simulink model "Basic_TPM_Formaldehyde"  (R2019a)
settings: Solver=ode15s  StartTime=0.0  StopTime=tend  RelTol=1e-3
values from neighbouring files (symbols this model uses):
  c_MeOH_0 = m_MeOH_sp_0/(m_MeOH_sp_0+m_air_sp_0)    [Mixer_script.m]
  comp_actuator_0 = [z0actuator,comp_w0]    [Compressor_script.m]
  comp_actuator_par = [comp_act_Ga;comp_act_tau;comp_act_zeta]    [Compressor_script.m]
  comp_deltaP = 2.1    [Compressor_script.m]
  comp_p1 = [a0,a1,a2,a3,b0,b1,b2,c0,c1,c2]    [Compressor_script.m]
  comp_p2 = [rho_a, kappa_a, cp_a, R_a, T_amb, d_c]    [Compressor_script.m]
  I_0_compressor = 0.39275    [Compressor_script.m]
  I_0_valve = valve_z0/valve_act_Ga    (= 0.7)    [Valve_script.m]
  Kc_comp = tau_compfotd/(K_compfotd*(tauc_comp+theta_compfotd))    [Compressor_script.m]
  Kc_mtot_air = tau_mtot_air/(K_mtot_air*(tauc_mtot_air+theta_mtot_air))    (= 0.512420362808)    [Basic_outer_PID_script.m]
  Kc_valve = tau_valvefotd/(K_valvefotd*(tauc_valve+theta_valvefotd))    [Valve_script.m]
  Kc_x_MeOH = tau_x_MeOH/(K_x_MeOH*(tauc_x_MeOH+theta_x_MeOH))    (= 21795.1661228)    [Basic_outer_PID_script.m]
  KI_comp = Kc_comp/tauI_comp    [Compressor_script.m]
  KI_mtot_air = Kc_mtot_air/tauI_mtot_air    [Basic_outer_PID_script.m]
  KI_valve = Kc_valve/tauI_valve    [Valve_script.m]
  KI_x_MeOH = Kc_x_MeOH/tauI_x_MeOH    [Basic_outer_PID_script.m]
  m_air_sp_0 = 23920    [Compressor_script.m]
  m_air_sp_step = m_air_sp_0*0*0.05    [main_basicTPM_formaldehyde.m]    (also in main_VPC_formaldehyde.m = m_air_sp_0*0; main_basic_formaldehyde.m = m_air_sp_0*0; main_SRC_formaldehyde.m = m_air_sp_0*0)
  m_air_sp_step_time = 20    [main_basicTPM_formaldehyde.m]    (also in main_VPC_formaldehyde.m; main_basic_formaldehyde.m; main_SRC_formaldehyde.m)
  m_MeOH_sp_0 = 2940    [Valve_script.m]
  m_MeOH_sp_step = -m_MeOH_sp_0*0.1    [main_basicTPM_formaldehyde.m]    (also in main_VPC_formaldehyde.m; main_basic_formaldehyde.m; main_SRC_formaldehyde.m)
  m_MeOH_sp_step_time = 20    [main_basicTPM_formaldehyde.m]    (also in main_VPC_formaldehyde.m; main_basic_formaldehyde.m; main_SRC_formaldehyde.m)
  m_tot_sp_0 = m_air_sp_0+m_MeOH_sp_0    [main_basicTPM_formaldehyde.m]    (also in main_VPC_formaldehyde.m; main_basic_formaldehyde.m; main_SRC_formaldehyde.m)
  m_tot_sp_step1 = 0*m_tot_sp_0*0.15    [main_basicTPM_formaldehyde.m]    (also in main_VPC_formaldehyde.m; main_basic_formaldehyde.m; main_SRC_formaldehyde.m)
  m_tot_sp_step2 = 1*m_tot_sp_0*0.10    [main_basicTPM_formaldehyde.m]    (also in main_VPC_formaldehyde.m; main_basic_formaldehyde.m; main_SRC_formaldehyde.m)
  m_tot_sp_step3 = -1*(m_tot_sp_step2+m_tot_sp_step1)    [main_basicTPM_formaldehyde.m]    (also in main_VPC_formaldehyde.m = 0*(m_tot_sp_step2+m_tot_sp_step1); main_basic_formaldehyde.m; main_SRC_formaldehyde.m)
  m_tot_sp_step_t1 = 20    [main_basicTPM_formaldehyde.m]    (also in main_VPC_formaldehyde.m; main_basic_formaldehyde.m; main_SRC_formaldehyde.m)
  m_tot_sp_step_t2 = 30    [main_basicTPM_formaldehyde.m]    (also in main_VPC_formaldehyde.m; main_basic_formaldehyde.m; main_SRC_formaldehyde.m)
  m_tot_sp_step_t3 = 70    [main_basicTPM_formaldehyde.m]    (also in main_VPC_formaldehyde.m = 60; main_basic_formaldehyde.m; main_SRC_formaldehyde.m)
  max_air_PI = mair_max-m_air_sp_0    [Basic_outer_PID_script.m]
  max_MeOH_PI = m_MeOH_max-m_MeOH_sp_0    [Basic_outer_PID_script.m]
  min_air_PI = mair_min-m_air_sp_0    [Basic_outer_PID_script.m]
  min_MeOH_PI = m_MeOH_min-m_MeOH_sp_0    [Basic_outer_PID_script.m]
  N_cmax = 10048    [Compressor_script.m]
  N_cmin = 7500    [Compressor_script.m]
  p_mix = [MW_MeOH;MW_air;rho_MeOH;rho_a;V_mixer]    [Mixer_script.m]
  PI_comp_max = 0.2    [Compressor_script.m]
  PI_comp_min = -I_0_compressor    (= -0.39275)    [Compressor_script.m]
  valve_actuator_0 = [valve_z0 valve_w0]    [Valve_script.m]
  valve_actuator_par = [valve_act_Ga;valve_act_tau;valve_act_zeta]    [Valve_script.m]
  valve_Cv = m_MeOH_max/sqrt(valve_delta_p)    [Valve_script.m]
  valve_delta_p = 0.5    [Valve_script.m]
  valve_type = 3    [Valve_script.m]
  x_MeOH_sp_step1 = 1*-0.005    (= -0.005)    [main_basicTPM_formaldehyde.m]    (also in main_VPC_formaldehyde.m; main_basic_formaldehyde.m; main_SRC_formaldehyde.m)
  x_MeOH_sp_step2 = 0*-0.005    (= 0)    [main_basicTPM_formaldehyde.m]    (also in main_VPC_formaldehyde.m; main_basic_formaldehyde.m; main_SRC_formaldehyde.m)
  x_MeOH_sp_step3 = 0*+0.01    (= 0)    [main_basicTPM_formaldehyde.m]    (also in main_VPC_formaldehyde.m; main_basic_formaldehyde.m; main_SRC_formaldehyde.m)
  x_MeOH_sp_step_t1 = 10    [main_basicTPM_formaldehyde.m]    (also in main_VPC_formaldehyde.m; main_basic_formaldehyde.m; main_SRC_formaldehyde.m)
  x_MeOH_sp_step_t2 = 40    [main_basicTPM_formaldehyde.m]    (also in main_VPC_formaldehyde.m; main_basic_formaldehyde.m; main_SRC_formaldehyde.m)
  x_MeOH_sp_step_t3 = 70    [main_basicTPM_formaldehyde.m]    (also in main_VPC_formaldehyde.m = 60; main_basic_formaldehyde.m; main_SRC_formaldehyde.m)
  x_MeOHsp_0 = 0.1    [main_basicTPM_formaldehyde.m]    (also in main_VPC_formaldehyde.m; main_basic_formaldehyde.m; main_SRC_formaldehyde.m)
undefined symbols (not defined in the file or in its folder): actuator, compressor, mixerMeOH_O2_dynamic, mixerMeOH_O2_ss, valve
libraries: simulink x4

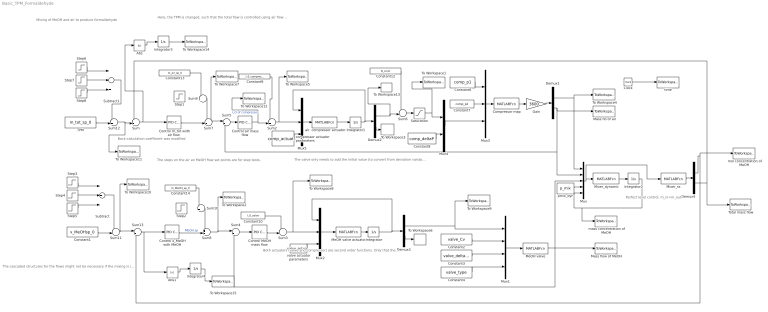
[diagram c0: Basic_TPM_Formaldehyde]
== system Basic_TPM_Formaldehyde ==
  note: Mixing of MeOH and air to produce formaldehyde
  note: The cascaded structures for the flows might not be necessary if the mixing is instantaneous. I just added them to have a general structure. I also added a small residence time in the tank.
  note: Both actuators (valve and compressor) are second order functions. Only that the time constants and the damping factors are different.
  note: The valve only needs to add the initial value (to convert from deviation variables to actual variables "once" before the actuator. The compressor also needs it before the actuator because the range does not start in 0. (Maybe there is a better way to do this).
  note: Perfect level control. m_in=m_out
  note: The steps on the air an MeOH flow set points are for step tests.
  note: Here, the TPM is changed, such that the total flow is controlled using air flow and the concentration is set by the flow of MeOH
  note: Back-calculation coefficient was modified
  Abs : Abs
  Abs1 : Abs
  Clock : Clock
  Compressor map : MATLABFcn  MATLABFcn=compressor(u(1:10),u(11:16),u(17:18))  OutputDimensions=2
  Constant1 : Constant  Value=x_MeOHsp_0
  Constant10 : Constant  Value=I_0_valve
  Constant12 : Constant  Value=N_cmin
  Constant13 : Constant  Value=m_air_sp_0
  Constant14 : Constant  Value=m_MeOH_sp_0
  Constant2 : Constant  Value=valve_Cv
  Constant3 : Constant  Value=valve_delta_p
  Constant4 : Constant  Value=valve_type
  Constant6 : Constant  Value=comp_p1
  Constant7 : Constant  Value=comp_p2
  Constant8 : Constant  Value=comp_deltaP
  Constant9 : Constant  Value=I_0_compressor
  Control MeOH mass flow : simulink/Continuous/PID Controller  Controller=PI  Form=Parallel  TimeDomain=Continuous-time  SampleTime=-1  IntegratorMethod=Forward Euler  FilterMethod=Forward Euler  ControllerParametersSource=internal  P=Kc_valve  I=KI_valve  D=0  UseFilter=on  N=100  TunerSelectOption=Transfer Function Based (PID Tuner App)  InitialConditionSource=internal  InitialConditionForIntegrator=0  InitialConditionForFilter=0  DifferentiatorICPrevScaledInput=0  ExternalReset=none  TrackingMode=off  Kt=1  LimitOutput=on  UpperSaturationLimit=1-I_0_valve  LowerSaturationLimit=-I_0_valve  LinearizeAsGain=on  AntiWindupMode=back-calculation  Kb=1  POutMin=[]  POutMax=[]  IOutMin=[]  IOutMax=[]  DOutMin=[]  DOutMax=[]  NOutMin=[]  NOutMax=[]  SumOutMin=[]  SumOutMax=[]  SaturationOutMin=[]  SaturationOutMax=[]  PParamMin=[]  PParamMax=[]  IParamMin=[]  IParamMax=[]  DParamMin=[]  DParamMax=[]  NParamMin=[]  NParamMax=[]  KbParamMin=[]  KbParamMax=[]  KtParamMin=[]  KtParamMax=[]  KbOutMin=[]  KbOutMax=[]  KtOutMin=[]  KtOutMax=[]  IntegratorOutMin=[]  IntegratorOutMax=[]  FilterOutMin=[]  FilterOutMax=[]  SumI1OutMin=[]  SumI1OutMax=[]  SumI2OutMin=[]  SumI2OutMax=[]  SumI3OutMin=[]  SumI3OutMax=[]  SumI4OutMin=[]  SumI4OutMax=[]  SumDOutMin=[]  SumDOutMax=[]  DifferentiatorOutMin=[]  DifferentiatorOutMax=[]  FilterDiffOutCoefMin=[]  FilterDiffOutCoefMax=[]  ReciprocalOutMin=[]  ReciprocalOutMax=[]  SumDenOutMin=[]  SumDenOutMax=[]  SumNumOutMin=[]  SumNumOutMax=[]  DivideOutMin=[]  DivideOutMax=[]  IntegratorContinuousStateAttributes=''  IntegratorStateMustResolveToSignalObject=off  IntegratorRTWStateStorageClass=Auto  FilterContinuousStateAttributes=''  FilterStateMustResolveToSignalObject=off  FilterRTWStateStorageClass=Auto  ParallelPVariant=InternalParameters  IdealPVariant=Disabled  IVariant=InternalParameters  DVariant=Disabled  IntegratorVariant=Continuous  SatVariant=Enabled  AWVariant=BackCalculation  PCopyVariant=Disabled  TRVariant=Disabled  FdbkBlocksVariant=Forward  IdealPFdbkVariant=Disabled  SatFdbkVariant=Disabled  DerivativeFilterVariant=Disabled  NVariant=Disabled  NCopyVariant=Disabled_SignalSpec  FilterICVariant=Disabled  IntegratorICVariant=InternalICs  ExternalResetVariant=Disabled  TRSumVariant=Passthrough  SumFdbkVariant=Disabled  SumVariant=Sum_PI
  Control air mass flow : simulink/Continuous/PID Controller  Controller=PI  Form=Parallel  TimeDomain=Continuous-time  SampleTime=-1  IntegratorMethod=Forward Euler  FilterMethod=Forward Euler  ControllerParametersSource=internal  P=Kc_comp  I=KI_comp  D=0  UseFilter=on  N=100  TunerSelectOption=Transfer Function Based (PID Tuner App)  InitialConditionSource=internal  InitialConditionForIntegrator=0  InitialConditionForFilter=0  DifferentiatorICPrevScaledInput=0  ExternalReset=none  TrackingMode=off  Kt=1  LimitOutput=on  UpperSaturationLimit=PI_comp_max  LowerSaturationLimit=PI_comp_min  LinearizeAsGain=on  AntiWindupMode=back-calculation  Kb=1  POutMin=[]  POutMax=[]  IOutMin=[]  IOutMax=[]  DOutMin=[]  DOutMax=[]  NOutMin=[]  NOutMax=[]  SumOutMin=[]  SumOutMax=[]  SaturationOutMin=[]  SaturationOutMax=[]  PParamMin=[]  PParamMax=[]  IParamMin=[]  IParamMax=[]  DParamMin=[]  DParamMax=[]  NParamMin=[]  NParamMax=[]  KbParamMin=[]  KbParamMax=[]  KtParamMin=[]  KtParamMax=[]  KbOutMin=[]  KbOutMax=[]  KtOutMin=[]  KtOutMax=[]  IntegratorOutMin=[]  IntegratorOutMax=[]  FilterOutMin=[]  FilterOutMax=[]  SumI1OutMin=[]  SumI1OutMax=[]  SumI2OutMin=[]  SumI2OutMax=[]  SumI3OutMin=[]  SumI3OutMax=[]  SumI4OutMin=[]  SumI4OutMax=[]  SumDOutMin=[]  SumDOutMax=[]  DifferentiatorOutMin=[]  DifferentiatorOutMax=[]  FilterDiffOutCoefMin=[]  FilterDiffOutCoefMax=[]  ReciprocalOutMin=[]  ReciprocalOutMax=[]  SumDenOutMin=[]  SumDenOutMax=[]  SumNumOutMin=[]  SumNumOutMax=[]  DivideOutMin=[]  DivideOutMax=[]  IntegratorContinuousStateAttributes=''  IntegratorStateMustResolveToSignalObject=off  IntegratorRTWStateStorageClass=Auto  FilterContinuousStateAttributes=''  FilterStateMustResolveToSignalObject=off  FilterRTWStateStorageClass=Auto  ParallelPVariant=InternalParameters  IdealPVariant=Disabled  IVariant=InternalParameters  DVariant=Disabled  IntegratorVariant=Continuous  SatVariant=Enabled  AWVariant=BackCalculation  PCopyVariant=Disabled  TRVariant=Disabled  FdbkBlocksVariant=Forward  IdealPFdbkVariant=Disabled  SatFdbkVariant=Disabled  DerivativeFilterVariant=Disabled  NVariant=Disabled  NCopyVariant=Disabled_SignalSpec  FilterICVariant=Disabled  IntegratorICVariant=InternalICs  ExternalResetVariant=Disabled  TRSumVariant=Passthrough  SumFdbkVariant=Disabled  SumVariant=Sum_PI
  "Control m_tot wiith air flow " : simulink/Continuous/PID Controller  Controller=PI  Form=Parallel  TimeDomain=Continuous-time  SampleTime=-1  IntegratorMethod=Forward Euler  FilterMethod=Forward Euler  ControllerParametersSource=internal  P=Kc_mtot_air  I=KI_mtot_air  D=0  UseFilter=on  N=100  TunerSelectOption=Transfer Function Based (PID Tuner App)  InitialConditionSource=internal  InitialConditionForIntegrator=0  InitialConditionForFilter=0  DifferentiatorICPrevScaledInput=0  ExternalReset=none  TrackingMode=off  Kt=1  LimitOutput=on  UpperSaturationLimit=max_air_PI  LowerSaturationLimit=min_air_PI  LinearizeAsGain=on  AntiWindupMode=back-calculation  Kb=0.1  POutMin=[]  POutMax=[]  IOutMin=[]  IOutMax=[]  DOutMin=[]  DOutMax=[]  NOutMin=[]  NOutMax=[]  SumOutMin=[]  SumOutMax=[]  SaturationOutMin=[]  SaturationOutMax=[]  PParamMin=[]  PParamMax=[]  IParamMin=[]  IParamMax=[]  DParamMin=[]  DParamMax=[]  NParamMin=[]  NParamMax=[]  KbParamMin=[]  KbParamMax=[]  KtParamMin=[]  KtParamMax=[]  KbOutMin=[]  KbOutMax=[]  KtOutMin=[]  KtOutMax=[]  IntegratorOutMin=[]  IntegratorOutMax=[]  FilterOutMin=[]  FilterOutMax=[]  SumI1OutMin=[]  SumI1OutMax=[]  SumI2OutMin=[]  SumI2OutMax=[]  SumI3OutMin=[]  SumI3OutMax=[]  SumI4OutMin=[]  SumI4OutMax=[]  SumDOutMin=[]  SumDOutMax=[]  DifferentiatorOutMin=[]  DifferentiatorOutMax=[]  FilterDiffOutCoefMin=[]  FilterDiffOutCoefMax=[]  ReciprocalOutMin=[]  ReciprocalOutMax=[]  SumDenOutMin=[]  SumDenOutMax=[]  SumNumOutMin=[]  SumNumOutMax=[]  DivideOutMin=[]  DivideOutMax=[]  IntegratorContinuousStateAttributes=''  IntegratorStateMustResolveToSignalObject=off  IntegratorRTWStateStorageClass=Auto  FilterContinuousStateAttributes=''  FilterStateMustResolveToSignalObject=off  FilterRTWStateStorageClass=Auto  ParallelPVariant=InternalParameters  IdealPVariant=Disabled  IVariant=InternalParameters  DVariant=Disabled  IntegratorVariant=Continuous  SatVariant=Enabled  AWVariant=BackCalculation  PCopyVariant=Disabled  TRVariant=Disabled  FdbkBlocksVariant=Forward  IdealPFdbkVariant=Disabled  SatFdbkVariant=Disabled  DerivativeFilterVariant=Disabled  NVariant=Disabled  NCopyVariant=Disabled_SignalSpec  FilterICVariant=Disabled  IntegratorICVariant=InternalICs  ExternalResetVariant=Disabled  TRSumVariant=Passthrough  SumFdbkVariant=Disabled  SumVariant=Sum_PI
  Control x_MeOH with MeOH : simulink/Continuous/PID Controller  Controller=PI  Form=Parallel  TimeDomain=Continuous-time  SampleTime=-1  IntegratorMethod=Forward Euler  FilterMethod=Forward Euler  ControllerParametersSource=internal  P=Kc_x_MeOH  I=KI_x_MeOH  D=0  UseFilter=on  N=100  TunerSelectOption=Transfer Function Based (PID Tuner App)  InitialConditionSource=internal  InitialConditionForIntegrator=0  InitialConditionForFilter=0  DifferentiatorICPrevScaledInput=0  ExternalReset=none  TrackingMode=off  Kt=1  LimitOutput=on  UpperSaturationLimit=max_MeOH_PI  LowerSaturationLimit=min_MeOH_PI  LinearizeAsGain=on  AntiWindupMode=back-calculation  Kb=1  POutMin=[]  POutMax=[]  IOutMin=[]  IOutMax=[]  DOutMin=[]  DOutMax=[]  NOutMin=[]  NOutMax=[]  SumOutMin=[]  SumOutMax=[]  SaturationOutMin=[]  SaturationOutMax=[]  PParamMin=[]  PParamMax=[]  IParamMin=[]  IParamMax=[]  DParamMin=[]  DParamMax=[]  NParamMin=[]  NParamMax=[]  KbParamMin=[]  KbParamMax=[]  KtParamMin=[]  KtParamMax=[]  KbOutMin=[]  KbOutMax=[]  KtOutMin=[]  KtOutMax=[]  IntegratorOutMin=[]  IntegratorOutMax=[]  FilterOutMin=[]  FilterOutMax=[]  SumI1OutMin=[]  SumI1OutMax=[]  SumI2OutMin=[]  SumI2OutMax=[]  SumI3OutMin=[]  SumI3OutMax=[]  SumI4OutMin=[]  SumI4OutMax=[]  SumDOutMin=[]  SumDOutMax=[]  DifferentiatorOutMin=[]  DifferentiatorOutMax=[]  FilterDiffOutCoefMin=[]  FilterDiffOutCoefMax=[]  ReciprocalOutMin=[]  ReciprocalOutMax=[]  SumDenOutMin=[]  SumDenOutMax=[]  SumNumOutMin=[]  SumNumOutMax=[]  DivideOutMin=[]  DivideOutMax=[]  IntegratorContinuousStateAttributes=''  IntegratorStateMustResolveToSignalObject=off  IntegratorRTWStateStorageClass=Auto  FilterContinuousStateAttributes=''  FilterStateMustResolveToSignalObject=off  FilterRTWStateStorageClass=Auto  ParallelPVariant=InternalParameters  IdealPVariant=Disabled  IVariant=InternalParameters  DVariant=Disabled  IntegratorVariant=Continuous  SatVariant=Enabled  AWVariant=BackCalculation  PCopyVariant=Disabled  TRVariant=Disabled  FdbkBlocksVariant=Forward  IdealPFdbkVariant=Disabled  SatFdbkVariant=Disabled  DerivativeFilterVariant=Disabled  NVariant=Disabled  NCopyVariant=Disabled_SignalSpec  FilterICVariant=Disabled  IntegratorICVariant=InternalICs  ExternalResetVariant=Disabled  TRSumVariant=Passthrough  SumFdbkVariant=Disabled  SumVariant=Sum_PI
  Demux{1..4} (4 alike) : Demux  Outputs=2
  Gain : Gain  Gain=3600
  Integrator : Integrator  InitialCondition=valve_actuator_0
  Integrator1 : Integrator  InitialCondition=comp_actuator_0
  Integrator2 : Integrator  InitialCondition=c_MeOH_0
  Integrator3 : Integrator
  Integrator4 : Integrator
  Mass flo of air : ToWorkspace  VariableName=m_air  SampleTime=-1
  Mass flow of MeOH : ToWorkspace  VariableName=m_MeOH  SampleTime=-1
  MeOH valve : MATLABFcn  MATLABFcn=valve(u)  OutputDimensions=1
  MeOH valve actuator : MATLABFcn  MATLABFcn=actuator(u(1:2),u(3),u(4:6))  OutputDimensions=2
  Mixer_dynamic : MATLABFcn  MATLABFcn=mixerMeOH_O2_dynamic(u(1:3),u(4:8),u(9))  OutputDimensions=1
  Mixer_ss : MATLABFcn  MATLABFcn=mixerMeOH_O2_ss(u(1:3),u(4:8),u(9))  OutputDimensions=2
  Mux : Mux  Inputs=5
  Mux1 : Mux
  Mux2 : Mux  Inputs=3
  Mux3 : Mux  Inputs=3
  Mux4 : Mux  Inputs=2
  Mux5 : Mux  Inputs=3
  Saturation : Saturate  UpperLimit=N_cmax  LowerLimit=N_cmin
  Step1 : Step  Time=m_air_sp_step_time  After=m_air_sp_step  SampleTime=0
  Step2 : Step  Time=m_MeOH_sp_step_time  After=m_MeOH_sp_step  SampleTime=0
  Step3 : Step  Time=x_MeOH_sp_step_t1  After=x_MeOH_sp_step1  SampleTime=0
  Step4 : Step  Time=x_MeOH_sp_step_t2  After=x_MeOH_sp_step2  SampleTime=0
  Step5 : Step  Time=x_MeOH_sp_step_t3  After=x_MeOH_sp_step3  SampleTime=0
  Step6 : Step  Time=m_tot_sp_step_t1  After=m_tot_sp_step1  SampleTime=0
  Step7 : Step  Time=m_tot_sp_step_t2  After=m_tot_sp_step2  SampleTime=0
  Step8 : Step  Time=m_tot_sp_step_t3  After=m_tot_sp_step3  SampleTime=0
  Subtract : Sum  Inputs=+++
  Subtract1 : Sum  Inputs=+++
  Sum : Sum  Inputs=-+|
  Sum{2..3,6..12} (9 alike) : Sum  Inputs=++|
  Sum13 : Sum  Inputs=|+-
  Sum4 : Sum  Inputs=|+-
  Sum5 : Sum  Inputs=|+-
  TPM : Constant  Value=m_tot_sp_0
  To Workspace1 : ToWorkspace  VariableName=comp_rpm  SampleTime=-1
  To Workspace10 : ToWorkspace  VariableName=x_MeOHsp  SampleTime=-1
  To Workspace11 : ToWorkspace  VariableName=m_tot_sp  SampleTime=-1
  To Workspace12 : ToWorkspace  VariableName=I_air0  SampleTime=-1
  To Workspace13 : ToWorkspace  VariableName=Nc_act  SampleTime=-1
  To Workspace14 : ToWorkspace  VariableName=IAExMeOH  SampleTime=-1
  To Workspace15 : ToWorkspace  VariableName=IAEmtot  SampleTime=-1
  To Workspace2 : ToWorkspace  VariableName=m_MEOH_sp  SampleTime=-1
  To Workspace3 : ToWorkspace  VariableName=wcomp  SampleTime=-1
  To Workspace4 : ToWorkspace  VariableName=Q_air  SampleTime=-1
  To Workspace5 : ToWorkspace  VariableName=I_air  SampleTime=-1
  To Workspace6 : ToWorkspace  VariableName=wvalve  SampleTime=-1
  To Workspace7 : ToWorkspace  VariableName=m_air_sp  SampleTime=-1
  To Workspace8 : ToWorkspace  VariableName=I_MeOH  SampleTime=-1
  To Workspace9 : ToWorkspace  VariableName=z_MeOH  SampleTime=-1
  Total mass flow : ToWorkspace  VariableName=m_tot  SampleTime=-1
  air  compressor actuator : MATLABFcn  MATLABFcn=actuator(u(1:2),u(3),u(4:6))  OutputDimensions=2
  compressor actuator parameters : Constant  Value=comp_actuator_par
  mass concentration of MeOH : ToWorkspace  VariableName=c_MeOH  SampleTime=-1
  mol concentration of MeOH : ToWorkspace  VariableName=x_MeOH  SampleTime=-1
  pmix_dyn : Constant  Value=p_mix
  time : ToWorkspace  VariableName=t  SampleTime=-1
  valve actuator parameters : Constant  Value=valve_actuator_par
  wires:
  MeOH valve/1 -> Mux/3, Mass flow of MeOH/1, Sum4/2
  Clock/1 -> time/1
  Mux1/1 -> MeOH valve/1
  Constant2/1 -> Mux1/2
  Constant3/1 -> Mux1/3
  Constant4/1 -> Mux1/4
  MeOH valve actuator/1 -> Integrator/1
  Mux2/1 -> MeOH valve actuator/1
  Integrator/1 -> Demux3/1, Mux2/1
  valve actuator parameters/1 -> Mux2/3
  Constant7/1 -> Mux3/2
  Constant6/1 -> Mux3/1
  Demux1/2 -> Mux/2, Sum5/2, Mass flo of air/1
  Demux1/1 -> To Workspace4/1, Mux/1
  Mux3/1 -> Compressor map/1
  Mux4/1 -> Mux3/3
  Constant8/1 -> Mux4/2
  Control air mass flow/1 -> Sum2/2, To Workspace12/1  "I_O of compressor"
  Constant9/1 -> Sum2/1
  Control MeOH mass flow/1 -> Sum3/2
  Sum3/1 -> To Workspace8/1, Mux2/2
  Constant10/1 -> Sum3/1
  air  compressor actuator/1 -> Integrator1/1
  Mux5/1 -> air  compressor actuator/1
  Integrator1/1 -> Demux2/1, Mux5/1
  Sum2/1 -> To Workspace5/1, Mux5/2
  compressor actuator parameters/1 -> Mux5/3
  Demux2/2 -> To Workspace3/1
  Demux3/2 -> To Workspace6/1
  Demux3/1 -> To Workspace9/1, Mux1/1
  Sum4/1 -> Control MeOH mass flow/1
  Sum5/1 -> Control air mass flow/1
  Sum/1 -> Abs/1, "Control m_tot wiith air flow "/1
  Sum6/1 -> Saturation/1
  Constant12/1 -> Sum6/1
  Saturation/1 -> To Workspace1/1, Mux4/1
  Demux2/1 -> To Workspace13/1, Sum6/2
  Gain/1 -> Demux1/1
  Compressor map/1 -> Gain/1
  Sum7/1 -> To Workspace7/1, Sum5/1
  Sum8/1 -> To Workspace2/1, Sum4/1
  Demux4/2 -> Total mass flow/1, Sum/1
  Constant13/1 -> Sum9/1
  Sum9/1 -> Sum7/1
  Demux4/1 -> mol concentration of MeOH/1, Sum13/2
  pmix_dyn/1 -> Mux/4
  Mux/1 -> Mixer_ss/1, Mixer_dynamic/1
  Mixer_dynamic/1 -> Integrator2/1
  Integrator2/1 -> mass concentration of MeOH/1, Mux/5
  Mixer_ss/1 -> Demux4/1
  Constant14/1 -> Sum10/1
  Sum10/1 -> Sum8/1
  Constant1/1 -> Sum11/2
  Sum11/1 -> Sum13/1, To Workspace10/1
  Subtract/1 -> Sum11/1
  Step3/1 -> Subtract/1
  Step4/1 -> Subtract/2
  Step5/1 -> Subtract/3
  TPM/1 -> Sum12/2
  Sum12/1 -> Sum/2, To Workspace11/1
  Step6/1 -> Subtract1/1
  Step7/1 -> Subtract1/2
  Step8/1 -> Subtract1/3
  Subtract1/1 -> Sum12/1
  Sum13/1 -> Control x_MeOH with MeOH/1, Abs1/1
  Control x_MeOH with MeOH/1 -> Sum8/2  "MEOH sp"
  "Control m_tot wiith air flow "/1 -> Sum7/2
  Abs/1 -> Integrator3/1
  Abs1/1 -> Integrator4/1
  Integrator3/1 -> To Workspace14/1
  Integrator4/1 -> To Workspace15/1
